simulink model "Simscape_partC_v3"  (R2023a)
settings: Solver=VariableStepAuto  StartTime=0.0  StopTime=10  FixedStep=1/(490*4)  RelTol=1e-3
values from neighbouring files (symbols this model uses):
  Kp = 250    [project_constants.m]
  theta_des = pi/2    (= 1.57079632679)    [project_constants.m]
libraries: fl_lib x7, nesl_utility x6, ee_lib x4, simulink x2

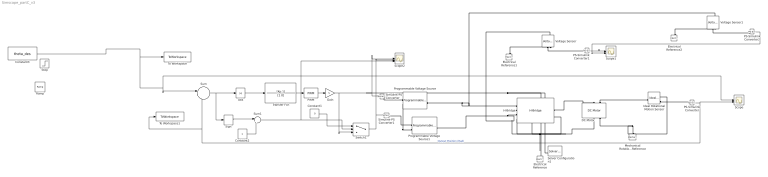
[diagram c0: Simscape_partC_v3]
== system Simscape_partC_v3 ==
  Abs : Abs
  Constant1 : Constant  Value=0
  Constant2 : Constant
  Constant3 : Constant  Value=theta_des
  DC Motor : ee_lib/Electromechanical/Brushed Motors/DC Motor  field_option=ee.enum.field_option.pm  Rf=100 Ohm  Lf=1 H  Laf=0.15 H  If0=0 A  parameterization=ee.enum.dcparam_option.circuit_param  Ra=5 Ohm  La=12e-6 H  emf_or_torque=ee.enum.emf_or_torque.ki  Kv=6/35 V/rpm  Ki=.1032 N*m/A  T_stall=140*9.81/1000 N*m  w_max=35 rpm  w_rated=15000 rpm  P_rated=0.08 W  V_rated=6 V  lam_param=ee.enum.lam_param.damping  i_noload=0 A  V_i_noload=1.5 V  J=9.76e-3 kg*m^2  lam=b N*m*s/rad  speed0=0 rpm  enable_fault_armature=simscape.enum.onoff.off  rev_faulted=1 / 3  G_faulted_armature=1e-5 S  fault_trigger_armature=ee.enum.faults.faultTrigger.temporal  t_fault_armature=1 s  max_permissible_current_armature=inf A  t_fail_on_current_armature=1 s  enable_fault_field=simscape.enum.onoff.off  G_faulted_field=1e-5 S  fault_trigger_field=ee.enum.faults.faultTrigger.temporal  t_fault_field=1 s  max_permissible_current_field=inf A  t_fail_on_current_field=1 s  fault_action=simscape.enum.assert.action.none  alpha=3.93e-3 1/K  Tmeas=25 degC  thermal_mass=100 J/K  initial_temperature=25 degC
  Electrical Reference : fl_lib/Electrical/Electrical Elements/Electrical Reference
  Electrical Reference1 : fl_lib/Electrical/Electrical Elements/Electrical Reference
  Electrical Reference2 : fl_lib/Electrical/Electrical Elements/Electrical Reference
  Gain : Gain  Gain=5
  H-Bridge : ee_lib/Semiconductors & Converters/Converters/H-Bridge  supply_ports=ee.enum.supply_ports.hidesupply  pwm_or_av=ee.enum.pwm_or_av.averaged  regenerative_braking_mode=ee.enum.converters.regenerative_braking_mode.depends_on_rev  discontinuous=ee.enum.current_profile.continuous  freewheeling_mode=ee.enum.converters.freewheeling_mode.one_switch_one_diode  Rload=10 Ohm  Lload=1e-5 H  F=10 kHz  Venable=2.5 V  Vmax=5 V  Vreverse=.1 V  Vbrake=.1 V  Vm=7.5 V  Ron=0.1 Ohm  Don=0.05 Ohm  Goff=1e-6 S  Tmeas=298.15 K  Ron2=0.1 Ohm  Don2=0.05 Ohm  Tmeas2=398.15 K  thermal_mass=100 J/K  initial_temperature=298.15 K
  Ideal Rotational Motion Sensor : fl_lib/Mechanical/Mechanical Sensors/Ideal Rotational Motion Sensor  reference=foundation.enum.MeasurementReference.difference  acceleration_port=false  velocity_port=true  position_port=true  wrap_angle=false  offset=0 rad
  Mechanical Rotational Reference : fl_lib/Mechanical/Rotational Elements/Mechanical Rotational Reference
  PS-Simulink Converter : nesl_utility/PS-Simulink Converter  PhysicalDomain=network_engine_domain  SubClassName=ps_output  LeftPortType=input  RightPortType=output  PseudoPeriodic=off  Frequencies=[]  VectorFormat=inherit  Unit=inherit  AffineConversion=off
  PS-Simulink Converter1 : nesl_utility/PS-Simulink Converter  PhysicalDomain=network_engine_domain  SubClassName=ps_output  LeftPortType=input  RightPortType=output  PseudoPeriodic=off  Frequencies=[]  VectorFormat=inherit  Unit=inherit  AffineConversion=off
  PS-Simulink Converter2 : nesl_utility/PS-Simulink Converter  PhysicalDomain=network_engine_domain  SubClassName=ps_output  LeftPortType=input  RightPortType=output  PseudoPeriodic=off  Frequencies=[]  VectorFormat=inherit  Unit=inherit  AffineConversion=off
  PWM : simulink/Discontinuities/PWM  DisableCoverage=on  Period=1/490  InitialDelay=0  DisallowZeroDutyCycle=off  RunAtFixedTimeIntervals=off  SampleTime=0.1
  Programmable Voltage Source : ee_lib/Sources/Programmable Voltage Source  magnitude_type=ee.enum.timechanging.constant  ac_magnitude=0 V  magn_ramp=1 V/s  magn_step=1 V  magn_modu_magn=1 V  magn_modu_freq=1 Hz  magn_t1=1 s  magn_t2=2 s  frequency_type=ee.enum.timechanging.constant  ac_frequency=60 Hz  freq_ramp=1 Hz/s  freq_step=1 Hz  freq_modu_magn=1 Hz  freq_modu_freq=1 Hz  freq_t1=1 s  freq_t2=2 s  phase_type=ee.enum.timechanging.constant  ac_shift=0 deg  phase_ramp=1 deg/s  phase_step=1 deg  phase_modu_magn=1 deg  phase_modu_freq=1 Hz  phase_t1=1 s  phase_t2=2 s  dc_type=ee.enum.timechanging.external  dc_voltage=0 V  dc_ramp=1 V/s  dc_step=1 V  dc_modu_magn=1 V  dc_modu_freq=1 Hz  dc_t1=1 s  dc_t2=2 s  harmonic_option=0  harmonic_orders=[5, 7, 11, 13]  harmonic_ratios=[.1, .1, .1, .1]  harmonic_shifts=[0, 0, 0, 0] deg  harmonic_t1=-inf s  harmonic_t2=inf s  noise_mode=0  PSD=0 V^2/Hz  repeatability=1  auto_seed=0  user_seed=0  sample_time=1e-3 s  i_specify=off  i_priority=None  i=0 A  i_nominal_specify=off  i_nominal_unit=A  i_nominal_value=1  v_specify=off  v_priority=None  v=0 V  v_nominal_specify=off  v_nominal_unit=V  v_nominal_value=1
  Programmable Voltage Source1 : ee_lib/Sources/Programmable Voltage Source  magnitude_type=ee.enum.timechanging.constant  ac_magnitude=0 V  magn_ramp=1 V/s  magn_step=1 V  magn_modu_magn=1 V  magn_modu_freq=1 Hz  magn_t1=1 s  magn_t2=2 s  frequency_type=ee.enum.timechanging.constant  ac_frequency=60 Hz  freq_ramp=1 Hz/s  freq_step=1 Hz  freq_modu_magn=1 Hz  freq_modu_freq=1 Hz  freq_t1=1 s  freq_t2=2 s  phase_type=ee.enum.timechanging.constant  ac_shift=0 deg  phase_ramp=1 deg/s  phase_step=1 deg  phase_modu_magn=1 deg  phase_modu_freq=1 Hz  phase_t1=1 s  phase_t2=2 s  dc_type=ee.enum.timechanging.external  dc_voltage=0 V  dc_ramp=1 V/s  dc_step=1 V  dc_modu_magn=1 V  dc_modu_freq=1 Hz  dc_t1=1 s  dc_t2=2 s  harmonic_option=0  harmonic_orders=[5, 7, 11, 13]  harmonic_ratios=[.1, .1, .1, .1]  harmonic_shifts=[0, 0, 0, 0] deg  harmonic_t1=-inf s  harmonic_t2=inf s  noise_mode=0  PSD=0 V^2/Hz  repeatability=1  auto_seed=0  user_seed=0  sample_time=1e-3 s  i_specify=off  i_priority=None  i=0 A  i_nominal_specify=off  i_nominal_unit=A  i_nominal_value=1  v_specify=off  v_priority=None  v=0 V  v_nominal_specify=off  v_nominal_unit=V  v_nominal_value=1
  Ramp : simulink/Sources/Ramp  slope=1  start=5  InitialOutput=pi/2
  Scope : Scope  NumInputPorts=2
  Scope1 : Scope  NumInputPorts=2
  Scope2 : Scope  NumInputPorts=3
  Sign : Signum
  Simulink-PS Converter : nesl_utility/Simulink-PS Converter  PhysicalDomain=network_engine_domain  SubClassName=ps_input  LeftPortType=input  RightPortType=output  PseudoPeriodic=off  Frequencies=[]  NoiseDistribution=none  NoiseParameters=[]  Unit=1  AffineConversion=off  FilteringAndDerivatives=provide  SimscapeFilterOrder=1  InputFilterTimeConstant=0.001  UdotUserProvided=0
  Simulink-PS Converter1 : nesl_utility/Simulink-PS Converter  PhysicalDomain=network_engine_domain  SubClassName=ps_input  LeftPortType=input  RightPortType=output  PseudoPeriodic=off  Frequencies=[]  NoiseDistribution=none  NoiseParameters=[]  Unit=1  AffineConversion=off  FilteringAndDerivatives=provide  SimscapeFilterOrder=1  InputFilterTimeConstant=0.001  UdotUserProvided=0
  Solver Configuration1 : nesl_utility/Solver Configuration  PhysicalDomain=network_engine_domain  SubClassName=solver  LeftPortType=input  RightPortType=generic  Tones=[]  Harmonics=[]  SimulateNoise=off  Profile=off  UseLocalSampling=off  EnableSwitchedLinearOptims=on  FrequencyDomain=off  UseCCode=off  RelTol=0.001  AbsTol=0.001  MinStep=1e-09  ToWorkspace=off  RevertToSquareIcSolve=off  NumHomotopyIterations=100  PhasorMode=off  PhasorModeNumHarmonics=1  ConsistencySolver=NEWTON_XTOL_AFTER_FTOL  IndexReductionMethod=DerivativeReplacement  DoDC=off  ResidualTolerance=1e-09  ConsistencyTolSource=GLOBAL  ConsistencyAbsTol=0.001  ConsistencyRelTol=0.001  ConsistencyTolFactor=0.001  UseLocalSolver=off  LocalSolverChoice=NE_BACKWARD_EULER_ADVANCER  ResolveIndetEquations=on  FunctionEvalNumThread=1  LocalSolverSampleTime=0.001  DoFixedCost=off  MaxNonlinIter=3  MaxModeIter=2  ComputeImpulses=off  ImpulseIterations=2  LinearAlgebra=auto  LinearAlgebraNumThread=0  EquationFormulation=NE_TIME_EF  DelaysMemoryBudget=1024  AutomaticFiltering=on  FilteringTimeConstant=0.001  PartitionStorageMethod=AS_NEEDED  PartitionMemoryBudget=1024  PartitionMethod=ROBUST
  Step : Step  Time=5  Before=pi/2  After=-pi/2  SampleTime=0
  Sum : Sum  Inputs=|+-
  Sum1 : Sum  Inputs=|++
  Switch1 : Switch  Criteria=u2 ~= 0
  To Workspace : ToWorkspace  VariableName=commanded_angle  SaveFormat=Structure With Time  SampleTime=-1
  To Workspace1 : ToWorkspace  VariableName=angle  SaveFormat=Structure With Time  SampleTime=-1
  Transfer Fcn : TransferFcn  Numerator=[Kp 1]  Denominator=[1 0]
  Voltage Sensor : fl_lib/Electrical/Electrical Sensors/Voltage Sensor
  Voltage Sensor1 : fl_lib/Electrical/Electrical Sensors/Voltage Sensor
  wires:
  PS-Simulink Converter/1 -> Scope/2, Sum/2, To Workspace1/1  "Output Position (Rad)"
  PS-Simulink Converter1/1 -> Scope1/1
  Constant3/1 -> Sum/1, Scope/1, To Workspace/1
  Abs/1 -> Transfer Fcn/1
  PWM/1 -> Gain/1
  Sum/1 -> Abs/1, Sign/1
  Transfer Fcn/1 -> PWM/1
  Gain/1 -> Simulink-PS Converter/1, Scope2/1, Switch1/3
  Switch1/1 -> Scope2/2, Simulink-PS Converter1/1
  Sign/1 -> Sum1/1
  Constant2/1 -> Sum1/2
  Sum1/1 -> Switch1/2, Scope2/3
  Constant1/1 -> Switch1/1
  PS-Simulink Converter2/1 -> Scope1/2
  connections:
  H-Bridge/RConn1 -- DC Motor/LConn1
  DC Motor/RConn2 -- Ideal Rotational Motion Sensor/RConn1 -- Mechanical Rotational Reference/LConn1
  DC Motor/LConn2 -- Ideal Rotational Motion Sensor/LConn1
  PS-Simulink Converter/LConn1 -- Ideal Rotational Motion Sensor/RConn3
  Programmable Voltage Source1/RConn2 -- Programmable Voltage Source/RConn2 -- H-Bridge/LConn2 -- H-Bridge/LConn4 -- DC Motor/RConn1 -- H-Bridge/RConn2 -- Solver Configuration1/RConn1 -- Electrical Reference/LConn1
  Programmable Voltage Source/LConn1 -- Voltage Sensor1/LConn1 -- H-Bridge/LConn1
  Programmable Voltage Source1/LConn1 -- Voltage Sensor/LConn1 -- H-Bridge/LConn3
  Electrical Reference1/LConn1 -- Voltage Sensor/RConn2
  Voltage Sensor/RConn1 -- PS-Simulink Converter1/LConn1
  Simulink-PS Converter/RConn1 -- Programmable Voltage Source/RConn1
  Simulink-PS Converter1/RConn1 -- Programmable Voltage Source1/RConn1
  Electrical Reference2/LConn1 -- Voltage Sensor1/RConn2
  Voltage Sensor1/RConn1 -- PS-Simulink Converter2/LConn1
